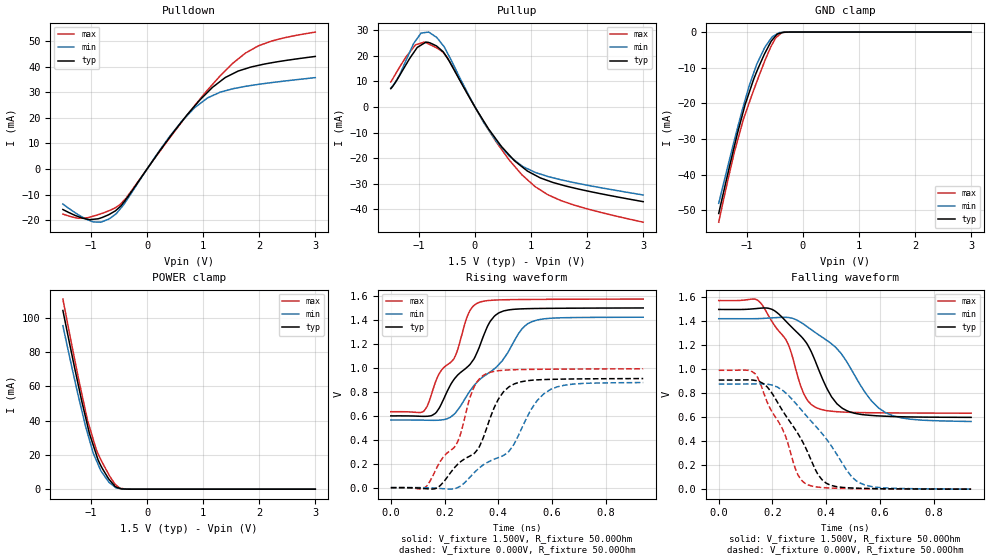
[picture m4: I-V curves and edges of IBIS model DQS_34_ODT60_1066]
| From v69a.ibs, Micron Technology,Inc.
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| MODEL DQS_34_ODT60_1066 (34 Ohm Data Strobe I/O with 60ohm ODT, 800/1066Mbps)
[Model]   DQS_34_ODT60_1066
Model_type   I/O
Vinl = 575.000mV
Vinh = 925.000mV
Vmeas = 750.000mV
Vref = 750.000mV
Cref = 0.0pF
Rref = 25.000Ohm
|   typ   min   max
C_comp   1.26pF   1.11pF   1.44pF
| Note: C_comp changes when the ODT circuit is enabled.
[Model Spec]
| Input threshold voltage corners
Vinl   0.5750V   0.5375V   0.6125V
Vinh   0.9250V   0.8875V   0.9625V
| Measurement voltage corners
Vmeas   0.7500V   0.7125V   0.7875V
| Timing spec test load voltage corners
Vref   0.7500V   0.7125V   0.7875V
|[Receiver Thresholds]
|Vth   =  0.750V
|Vth_min  =  0.735V
|Vth_max  =  0.765V
|Vinh_ac  =  0.175V
|Vinh_dc  =  0.100V
|Vinl_ac  = -0.175V
|Vinl_dc  = -0.100V
|Tslew_ac =  5.000ns |Not specified, so set to high value
|Threshold_sensitivity = 0.50
|Reference_supply Pullup_ref
[Receiver Thresholds]
Vcross_low   = 0.575V
Vcross_high  = 0.925V
Vdiff_ac   = 350mV
Vdiff_dc   = 200mV
Tdiffslew_ac = 10.000ns |Not specified, so set to high value
[Voltage Range]   1.5000V   1.4250V   1.5750V
[Pullup Reference]   1.5000V   1.4250V   1.5750V
| Junction Temperature (Ambient temp is 35C typ, 95C min, 0C max)
[Temperature Range]   50.0   110.0   0.0
[Add Submodel]
| Submodel Name   Mode
60ohm_ODT_1066   Non-Driving
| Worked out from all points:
|   slope of the pulldown table from 0 to 0.225 V, typ, clamps not added: 31.9 ohm
|   slope of the pullup table from 0 to 0.225 V, typ, clamps not added: 28.4 ohm
|   GND clamp passes 1 mA (typ) near -0.48 V on its own axis
|   POWER clamp passes 1 mA (typ) near -0.53 V on its own axis
|   falling waveform, V_fixture 1.500V, R_fixture 50.00Ohm: 20-80 % time 131ps typ, 173ps min, 110ps max; typ from 1.5 V to 0.599 V
|   rising waveform, V_fixture 1.500V, R_fixture 50.00Ohm: 20-80 % time 150ps typ, 192ps min, 121ps max; typ from 0.599 V to 1.5 V
|   rising waveform, V_fixture 0.000V, R_fixture 50.00Ohm: 20-80 % time 155ps typ, 202ps min, 123ps max; typ from 0 V to 0.911 V
|   falling waveform, V_fixture 0.000V, R_fixture 50.00Ohm: 20-80 % time 138ps typ, 179ps min, 112ps max; typ from 0.911 V to 0 V
[Pulldown]
|   Voltage   I(typ)   I(min)   I(max)
-1.5V     -15.86mA   -13.71mA   -17.64mA
-1.22V    -18.7mA    -17.99mA   -19.3mA
-965mV    -19.7mA    -20.68mA   -18.5mA
-680mV    -17.86mA   -19.62mA   -16.37mA
-375mV    -11.88mA   -12.6mA    -11.45mA
390mV     11.99mA    12.36mA    11.75mA
845mV     24.56mA    23.92mA    24.71mA
1.075V    29.95mA    27.78mA    30.82mA
1.395V    35.82mA    30.62mA    38.47mA
1.755V    39.25mA    32.36mA    45.39mA
1.985V    40.57mA    33.14mA    48.21mA
3V        44.07mA    35.78mA    53.61mA
[GND Clamp]
|   Voltage   I(typ)   I(min)   I(max)
-1.5V     -50.86mA   -48.03mA   -53.31mA
-1.335V   -39.51mA   -37.41mA   -41.36mA
-1.22V    -31.91mA   -30.23mA   -33.59mA
-1.06V    -22.14mA   -20.74mA   -24.46mA
-1.03V    -20.37mA   -19.08mA   -23.1mA
-960mV    -17.09mA   -15.22mA   -19.96mA
-825mV    -11.18mA   -9.113mA   -14.07mA
-680mV    -6.012mA   -4.321mA   -8.138mA
-565mV    -2.562mA   -1.714mA   -3.942mA
-485mV    -1.053mA   -743.8uA   -1.64mA
-380mV    -208.9uA   -97.58uA   -211uA
3V        0A         0A         0A
[Pullup]
|   Voltage   I(typ)   I(min)   I(max)
-1.5V     7.178mA    7.449mA    9.786mA
-1.34V    12.44mA    12.71mA    15.73mA
-1.06V    22.29mA    25.85mA    24.28mA
-960mV    24.22mA    28.89mA    24.98mA
-825mV    25.21mA    29.28mA    24.64mA
-680mV    23.76mA    27.16mA    23.08mA
-485mV    18.85mA    20.88mA    19.1mA
155mV     -5.461mA   -5.981mA   -5.833mA
615mV     -18.83mA   -19.23mA   -20.79mA
845mV     -23.43mA   -23.12mA   -26.61mA
1.525V    -30.28mA   -28.36mA   -36.46mA
3V        -36.95mA   -34.34mA   -44.97mA
[POWER Clamp]
|   Voltage   I(typ)   I(min)   I(max)
-1.5V     104.2mA    95.33mA    110.8mA
-1.22V    59.88mA    53.65mA    64.17mA
-1.06V    36.99mA    32.51mA    40.06mA
-1.025V   32.28mA    28.5mA     36.2mA
-960mV    25.75mA    21.1mA     29.08mA
-875mV    17.23mA    14.62mA    20.76mA
-825mV    13.81mA    10.81mA    17.3mA
-690mV    6.286mA    4.503mA    9.027mA
-565mV    1.438mA    1.112mA    2.719mA
-490mV    520.5uA    387uA      712uA
-290mV    1.769uA    1.056uA    286.1nA
3V        0A         0A         0A
[Ramp]
R_load = 50.00Ohm
|   typ   min   max
dV/dt_r   546.393mV/154.890ps 526.113mV/201.700ps 595.210mV/122.633ps
dV/dt_f   540.353mV/131.410ps 514.673mV/172.562ps 564.059mV/110.122ps
[Falling Waveform]
V_fixture = 1.500V
V_fixture_min = 1.425V
V_fixture_max = 1.575V
R_fixture = 50.00Ohm
|   Time   V(typ)   V(min)   V(max)
0s        1.5V       1.423V     1.574V
155ps     1.51V      1.424V     1.556V
235ps     1.437V     1.434V     1.292V
260ps     1.379V     1.433V     1.204V
320ps     1.24V      1.371V     781.6mV
365ps     1.038V     1.299V     678.3mV
460ps     675.3mV    1.12V      643.8mV
545ps     619.8mV    807.5mV    638.6mV
620ps     609mV      640.4mV    636.8mV
940ps     599.3mV    564.9mV    634mV
[Rising Waveform]
V_fixture = 1.500V
V_fixture_min = 1.425V
V_fixture_max = 1.575V
R_fixture = 50.00Ohm
|   Time   V(typ)   V(min)   V(max)
0s        599.3mV    564.9mV    634mV
125ps     595.3mV    563.4mV    644mV
170ps     630.2mV    562.6mV    902.8mV
220ps     848.1mV    584.9mV    1.041V
245ps     929.7mV    636.6mV    1.127V
290ps     1.017V     791.6mV    1.456V
320ps     1.123V     877.8mV    1.537V
390ps     1.44V      1V         1.566V
525ps     1.495V     1.385V     1.571V
940ps     1.5V       1.423V     1.574V
[Rising Waveform]
V_fixture = 0.000V
V_fixture_min = 0.000V
V_fixture_max = 0.000V
R_fixture = 50.00Ohm
|   Time   V(typ)   V(min)   V(max)
0s        -4.765uV   687.2uV    159.9uV
135ps     -9.198mV   -399.1uV   16.67mV
180ps     10.05mV    -5.873mV   203.6mV
250ps     197.9mV    2.227mV    388.1mV
310ps     284.4mV    124.1mV    840mV
360ps     516.8mV    211.6mV    955.1mV
440ps     841.6mV    304.3mV    982.9mV
525ps     896.7mV    661.3mV    987.3mV
595ps     904mV      820mV      988.8mV
940ps     910.7mV    877.5mV    992.2mV
[Falling Waveform]
V_fixture = 0.000V
V_fixture_min = 0.000V
V_fixture_max = 0.000V
R_fixture = 50.00Ohm
|   Time   V(typ)   V(min)   V(max)
0s        910.7mV    877.5mV    992.2mV
135ps     907.9mV    878.8mV    964.5mV
180ps     854.4mV    875.8mV    729.5mV
225ps     701.8mV    843.5mV    553mV
295ps     463.6mV    694.4mV    119.2mV
330ps     315.1mV    603.2mV    38.8mV
370ps     121.4mV    502.9mV    17.17mV
400ps     50.79mV    421.2mV    11.29mV
525ps     7.426mV    52.76mV    4.17mV
940ps     -4.765uV   687.2uV    159.9uV
